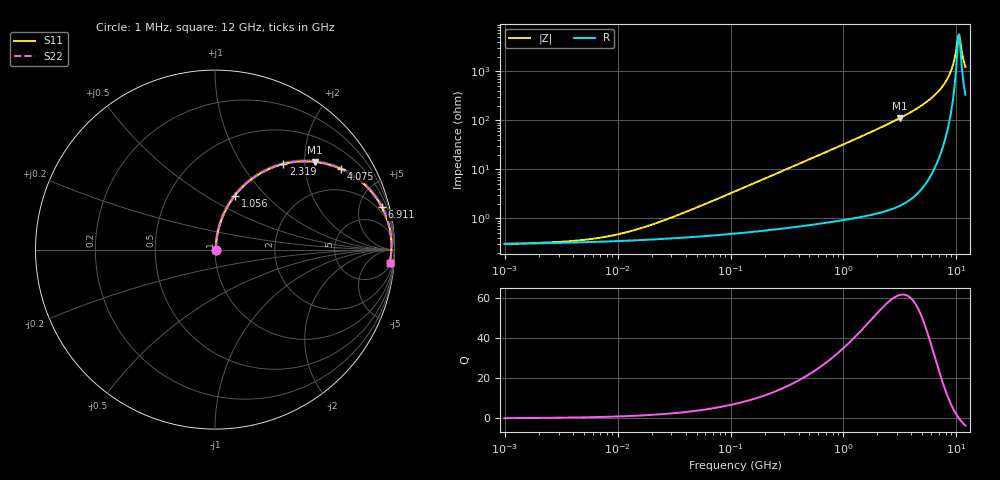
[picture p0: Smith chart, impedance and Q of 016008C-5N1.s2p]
# MHz S MA R 50
!Freq  MagS11  AngS11  MagS21  AngS21  MagS12  AngS12  MagS22  AngS22
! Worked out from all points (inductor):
!   801 points, 1 MHz to 12 GHz, reference 50 ohm
!   read as one part in series: L = 5.1 nH near 37.63 MHz
!   highest Q = 61.8 at 3.184 GHz (marker M1), where L = 5.62 nH
!   self-resonance near 10.42 GHz
!   S11 on the Smith chart (normalised r, x): 1 MHz: 1.01, +0.00; 1.056 GHz: 1.02, +0.68; 2.319 GHz: 1.03, +1.56; 4.075 GHz: 1.05, +3.07; 6.911 GHz: 1.31, +7.79; 12 GHz: 8, -24
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1  0.003006 6.1  0.997 -0.0  0.997 -0.0  0.003006 6.1
4.822396  0.003573 25.4  0.9968 -0.1  0.9968 -0.1  0.003573 25.4
10.46635  0.004788 44.1  0.9966 -0.2  0.9966 -0.2  0.004788 44.1
22.98406  0.008233 62.6  0.9962 -0.4  0.9962 -0.4  0.008233 62.6
110.8382  0.03566 80.1  0.9945 -2.0  0.9945 -2.0  0.03566 80.1
528.267  0.1663 77.9  0.9789 -9.6  0.9789 -9.6  0.1663 77.9
1056.071  0.3209 69.7  0.9383 -18.7  0.9383 -18.7  0.3209 69.7
1574.194  0.4547 61.7  0.8809 -27.0  0.8809 -27.0  0.4547 61.7
2319.127  0.6105 51.4  0.7813 -37.6  0.7813 -37.6  0.6105 51.4
2517.778  0.6449 48.9  0.7533 -40.2  0.7533 -40.2  0.6449 48.9
3184.175  0.7411 41.3  0.6595 -47.8  0.6595 -47.8  0.7411 41.3
4074.51  0.8318 32.8  0.5413 -56.3  0.5413 -56.3  0.8318 32.8
5464.492  0.9157 22.4  0.3816 -66.3  0.3816 -66.3  0.9157 22.4
6910.816  0.9594 14.2  0.2461 -73.5  0.2461 -73.5  0.9594 14.2
7956.408  0.9751 9.4  0.1638 -76.6  0.1638 -76.6  0.9751 9.4
8843.168  0.9816 5.8  0.1023 -76.8  0.1023 -76.8  0.9816 5.8
9377.838  0.9834 3.8  0.06858 -74.1  0.06858 -74.1  0.9834 3.8
10181.12  0.9835 1.1  0.0251 -48.4  0.0251 -48.4  0.9835 1.1
10423.02  0.983 0.3  0.01778 -17.4  0.01778 -17.4  0.983 0.3
10796.69  0.982 -0.9  0.02341 39.2  0.02341 39.2  0.982 -0.9
11584.69  0.9783 -3.2  0.05935 67.0  0.05935 67.0  0.9783 -3.2
12000  0.9757 -4.4  0.07905 70.0  0.07905 70.0  0.9757 -4.4
